| This Model is valid for Automotive grade 2 Temperature Range -40C<=Tc<=105C
| Valid for LPDDR4-4266 operation
| Part Number   VDD/VDDQ   Package   Architecture
| SCB11N4G160BF-04ZA2   1.1 +0.07/-0.04  BGA   4G bit x 16
[IBIS ver] 5.0
[File name]  usssn4g16ba2.ibs
[File Rev]  1.0
[Date]   October 8, 2023
[Source] Simulation of a silicon level SPICE model
[Notes]  IBIS Characteristics for I/O Buffer
  IBIS Model Revision History: Rev 1.0:
  2023-10-08 - IBIS model file initial creation
[Disclaimer]  The IBIS models are for modeling purpose only and are subject to change without any notice. UniIC is not
  responsible for any problems the models may cause.
[Copyright] Copyright 2023 UniIC Semiconductors Corp. All rights reserved
|   Component SCB11N4G160BF-04ZA2
[Component] SCB11N4G160BF-04ZA2
[Manufacturer] UniIC Semiconductors Corp.
[Package]
| variable   typ   min   max
R_pkg   0.750   0.698   0.832
L_pkg   1.500nH   1.330nH   1.720nH
C_pkg   0.630pF   0.579pF   0.668pF
[Pin]  signal_name   model_name   R_pin   L_pin   C_pin
A1   DNU   NC
A2   DNU   NC
A3   VSS   Gnd
A4   VDD2   Power
A5   ZQ0   NC
A8   NC   NC
A9   VDD2   Power
A10   VSS   Gnd
A11   DNU   NC
A12   DNU   NC
AA1   DNU   NC
AA2   NC   NC
AA3   VDDQ   Power
AA4   NC   NC
AA5   VDDQ   Power
AA8   VDDQ   Power
AA9   NC   NC
AA10   VDDQ   Power
AA11   NC   NC
AA12   DNU   NC
AB1   DNU   NC
AB2   DNU   NC
AB3   VSS   Gnd
AB4   VDD2   Power
AB5   VSS   Gnd
AB8   VSS   Gnd
AB9   VDD2   Power
AB10   VSS   Gnd
AB11   DNU   NC
AB12   DNU   NC
B1   DNU   NC
B2   DQ0_A   DQ   0.825   1.680nH   0.658pF
B3   VDDQ   Power
B4   DQ7_A   DQ   0.810   1.640nH   0.579pF
B5   VDDQ   Power
B8   VDDQ   Power
B9   DQ15_A   DQ   0.819   1.720nH   0.645pF
B10   VDDQ   Power
B11   DQ8_A   DQ   0.832   1.650nH   0.595pF
B12   DNU   NC
C1   VSS   Gnd
C2   DQ1_A   DQ   0.809   1.620nH   0.658pF
C3   DMI0_A   DQ   0.816   1.600nH   0.644pF
C4   DQ6_A   DQ   0.782   1.720nH   0.645pF
C5   VSS   Gnd
C8   VSS   Gnd
C9   DQ14_A   DQ   0.776   1.550nH   0.639pF
C10   DMI1_A   DQ   0.793   1.560nH   0.644pF
C11   DQ9_A   DQ   0.809   1.640nH   0.668pF
C12   VSS   Gnd
D1   VDDQ   Power
D2   VSS   Gnd
D3   DQS0_T_A   DQS   0.752   1.480nH   0.614pF
D4   VSS   Gnd
D5   VDDQ   Power
D8   VDDQ   Power
D9   VSS   Gnd
D10   DQS1_T_A   DQS   0.750   1.460nH   0.630pF
D11   VSS   Gnd
D12   VDDQ   Power
E1   VSS   Gnd
E2   DQ2_A   DQ   0.772   1.490nH   0.579pF
E3   DQS0_C_A   DQS   0.739   1.480nH   0.613pF
E4   DQ5_A   DQ   0.698   1.360nH   0.629pF
E5   VSS   Gnd
E8   VSS   Gnd
E9   DQ13_A   DQ   0.701   1.330nH   0.647pF
E10   DQS1_C_A   DQS   0.749   1.470nH   0.622pF
E11   DQ10_A   DQ   0.786   1.530nH   0.591pF
E12   VSS   Gnd
F1   VDD1   Power
F2   DQ3_A   DQ   0.748   1.480nH   0.582pF
F3   VDDQ   Power
F4   DQ4_A   DQ   0.740   1.430nH   0.640pF
F5   VDD2   Power
F8   VDD2   Power
F9   DQ12_A   DQ   0.751   1.420nH   0.664pF
F10   VDDQ   Power
F11   DQ11_A   DQ   0.765   1.520nH   0.562pF
F12   VDD1   Power
G1   VSS   Gnd
G2   ODTCA_A   RCV_RST_N
G3   VSS   Gnd
G4   VDD1   Power
G5   VSS   Gnd
G8   VSS   Gnd
G9   VDD1   Power
G10   VSS   Gnd
G11   NC   NC
G12   VSS   Gnd
H1   VDD2   Power
H2   CA0_A   CA   1.640   2.810nH   1.140pF
H3   NC   NC
H4   CS0_A   CA   1.170   2.210nH   0.905pF
H5   VDD2   Power
H8   VDD2   Power
H9   CA2_A   CA   1.550   2.690nH   1.150pF
H10   CA3_A   CA   1.570   2.740nH   1.120pF
H11   CA4_A   CA   1.600   2.780nH   1.160pF
H12   VDD2   Power
J1   VSS   Gnd
J2   CA1_A   CA   1.670   2.970nH   1.170pF
J3   VSS   Gnd
J4   CKE0_A   RCV_CKE   1.490   2.670nH   1.000pF
J5   NC   NC
J8   CKT_A   CLK   1.400   2.570nH   1.060pF
J9   CKC_A   CLK   1.420   2.610nH   1.070pF
J10   VSS   Gnd
J11   CA5_A   CA   1.710   2.940nH   1.200pF
J12   VSS   Gnd
K1   VDD2   Power
K2   VSS   Gnd
K3   VDD2   Power
K4   VSS   Gnd
K5   NC   NC
K8   NC   NC
K9   VSS   Gnd
K10   VDD2   Power
K11   VSS   Gnd
K12   VDD2   Power
N1   VDD2   Power
N2   VSS   Gnd
N3   VDD2   Power
N4   VSS   Gnd
N5   CS3_A   CA
N8   CKE3_A   RCV_CKE
N9   VSS   Gnd
N10   VDD2   Power
N11   VSS   Gnd
N12   VDD2   Power
P1   VSS   Gnd
P2   NC   NC
P3   VSS   Gnd
P4   NC   NC
P5   NC   NC
P8   NC   NC
P9   NC   NC
P10   VSS   Gnd
P11   NC   NC
P12   VSS   Gnd
R1   VDD2   Power
R2   NC   NC
R3   NC   NC
R4   NC   NC
R5   VDD2   Power
R8   VDD2   Power
R9   NC   NC
R10   NC   NC
R11   NC   NC
R12   VDD2   Power
T1   VSS   Gnd
T2   NC   NC
T3   VSS   Gnd
T4   VDD1   Power
T5   VSS   Gnd
T8   VSS   Gnd
T9   VDD1   Power
T10   VSS   Gnd
T11   RESET_N   RCV_RST_N
T12   VSS   Gnd
U1   VDD1   Power
U2   NC   NC
U3   VDDQ   Power
U4   NC   NC
U5   VDD2   Power
U8   VDD2   Power
U9   NC   NC
U10   VDDQ   Power
U11   NC   NC
U12   VDD1   Power
V1   VSS   Gnd
V2   NC   NC
V3   NC   NC
V4   NC   NC
V5   VSS   Gnd
V8   VSS   Gnd
V9   NC   NC
V10   NC   NC
V11   NC   NC
V12   VSS   Gnd
W1   VDDQ   Power
W2   VSS   Gnd
W3   NC   NC
W4   VSS   Gnd
W5   VDDQ   Power
W8   VDDQ   Power
W9   VSS   Gnd
W10   NC   NC
W11   VSS   Gnd
W12   VDDQ   Power
Y1   VSS   Gnd
Y2   NC   NC
Y3   NC   NC
Y4   NC   NC
Y5   VSS   Gnd
Y8   VSS   Gnd
Y9   NC   NC
Y10   NC   NC
Y11   NC   NC
Y12   VSS   Gnd
|IN   dq_in   dummy
|EN   dq_en   dummy
[Diff pin]  inv_pin  vdiff   tdelay_typ   tdelay_min   tdelay_max
D3   E3   0.160V   NA   NA   NA
D10   E10   0.160V   NA   NA   NA
J8   J9   0.160V   NA   NA   NA
[Model Selector] DQ
DQ_PU_PD_480_240_DRIVE_SOCODT240_VOH33  voh=vddq/3, 480 Ohm Pullup, 240 Ohm Pulldown,240ohm SOCODT
DQ_PU_PD_480_120_DRIVE_SOCODT240_VOH33  voh=vddq/3, 480 Ohm Pullup, 120 Ohm Pulldown,240ohm SOCODT
DQ_PU_PD_480_80_DRIVE_SOCODT240_VOH33  voh=vddq/3, 480 Ohm Pullup, 80 Ohm Pulldown,240ohm SOCODT
DQ_PU_PD_480_60_DRIVE_SOCODT240_VOH33  voh=vddq/3, 480 Ohm Pullup, 60 Ohm Pulldown,240ohm SOCODT
DQ_PU_PD_480_48_DRIVE_SOCODT240_VOH33  voh=vddq/3, 480 Ohm Pullup, 48 Ohm Pulldown,240ohm SOCODT
DQ_PU_PD_480_40_DRIVE_SOCODT240_VOH33  voh=vddq/3, 480 Ohm Pullup, 40 Ohm Pulldown,240ohm SOCODT
DQ_PU_PD_240_240_DRIVE_SOCODT120_VOH33  voh=vddq/3, 240 Ohm Pullup, 240 Ohm Pulldown,120ohm SOCODT
DQ_PU_PD_240_120_DRIVE_SOCODT120_VOH33  voh=vddq/3, 240 Ohm Pullup, 120 Ohm Pulldown,120ohm SOCODT
DQ_PU_PD_240_80_DRIVE_SOCODT120_VOH33  voh=vddq/3, 240 Ohm Pullup, 80 Ohm Pulldown,120ohm SOCODT
DQ_PU_PD_240_60_DRIVE_SOCODT120_VOH33  voh=vddq/3, 240 Ohm Pullup, 60 Ohm Pulldown,120ohm SOCODT
DQ_PU_PD_240_48_DRIVE_SOCODT120_VOH33  voh=vddq/3, 240 Ohm Pullup, 48 Ohm Pulldown,120ohm SOCODT
DQ_PU_PD_240_40_DRIVE_SOCODT120_VOH33  voh=vddq/3, 240 Ohm Pullup, 40 Ohm Pulldown,120ohm SOCODT
DQ_PU_PD_160_240_DRIVE_SOCODT80_VOH33  voh=vddq/3, 160 Ohm Pullup, 240 Ohm Pulldown,80ohm SOCODT
DQ_PU_PD_160_120_DRIVE_SOCODT80_VOH33  voh=vddq/3, 160 Ohm Pullup, 120 Ohm Pulldown,80ohm SOCODT
DQ_PU_PD_160_80_DRIVE_SOCODT80_VOH33  voh=vddq/3, 160 Ohm Pullup, 80 Ohm Pulldown,80ohm SOCODT
DQ_PU_PD_160_60_DRIVE_SOCODT80_VOH33  voh=vddq/3, 160 Ohm Pullup, 60 Ohm Pulldown,80ohm SOCODT
DQ_PU_PD_160_48_DRIVE_SOCODT80_VOH33  voh=vddq/3, 160 Ohm Pullup, 48 Ohm Pulldown,80ohm SOCODT
DQ_PU_PD_160_40_DRIVE_SOCODT80_VOH33  voh=vddq/3, 160 Ohm Pullup, 40 Ohm Pulldown,80ohm SOCODT
DQ_PU_PD_120_240_DRIVE_SOCODT60_VOH33  voh=vddq/3, 120 Ohm Pullup, 240 Ohm Pulldown,60ohm SOCODT
DQ_PU_PD_120_120_DRIVE_SOCODT60_VOH33  voh=vddq/3, 120 Ohm Pullup, 120 Ohm Pulldown,60ohm SOCODT
DQ_PU_PD_120_80_DRIVE_SOCODT60_VOH33  voh=vddq/3, 120 Ohm Pullup, 80 Ohm Pulldown,60ohm SOCODT
DQ_PU_PD_120_60_DRIVE_SOCODT60_VOH33  voh=vddq/3, 120 Ohm Pullup, 60 Ohm Pulldown,60ohm SOCODT
DQ_PU_PD_120_48_DRIVE_SOCODT60_VOH33  voh=vddq/3, 120 Ohm Pullup, 48 Ohm Pulldown,60ohm SOCODT
DQ_PU_PD_120_40_DRIVE_SOCODT60_VOH33  voh=vddq/3, 120 Ohm Pullup, 40 Ohm Pulldown,60ohm SOCODT
DQ_PU_PD_96_240_DRIVE_SOCODT48_VOH33  voh=vddq/3, 96 Ohm Pullup, 240 Ohm Pulldown,48ohm SOCODT
DQ_PU_PD_96_120_DRIVE_SOCODT48_VOH33  voh=vddq/3, 96 Ohm Pullup, 120 Ohm Pulldown,48ohm SOCODT
DQ_PU_PD_96_80_DRIVE_SOCODT48_VOH33  voh=vddq/3, 96 Ohm Pullup, 80 Ohm Pulldown,48ohm SOCODT
DQ_PU_PD_96_60_DRIVE_SOCODT48_VOH33  voh=vddq/3, 96 Ohm Pullup, 60 Ohm Pulldown,48ohm SOCODT
DQ_PU_PD_96_48_DRIVE_SOCODT48_VOH33  voh=vddq/3, 96 Ohm Pullup, 48 Ohm Pulldown,48ohm SOCODT
DQ_PU_PD_96_40_DRIVE_SOCODT48_VOH33  voh=vddq/3, 96 Ohm Pullup, 40 Ohm Pulldown,48ohm SOCODT
DQ_PU_PD_80_240_DRIVE_SOCODT40_VOH33  voh=vddq/3, 80 Ohm Pullup, 240 Ohm Pulldown,SOCODT disable OR 40ohm SOCODT
DQ_PU_PD_80_120_DRIVE_SOCODT40_VOH33  voh=vddq/3, 80 Ohm Pullup, 120 Ohm Pulldown,SOCODT disable OR 40ohm SOCODT
DQ_PU_PD_80_80_DRIVE_SOCODT40_VOH33  voh=vddq/3, 80 Ohm Pullup, 80 Ohm Pulldown,SOCODT disable OR 40ohm SOCODT
DQ_PU_PD_80_60_DRIVE_SOCODT40_VOH33  voh=vddq/3, 80 Ohm Pullup, 60 Ohm Pulldown,SOCODT disable OR 40ohm SOCODT
DQ_PU_PD_80_48_DRIVE_SOCODT40_VOH33  voh=vddq/3, 80 Ohm Pullup, 48 Ohm Pulldown,SOCODT disable OR 40ohm SOCODT
DQ_PU_PD_80_40_DRIVE_SOCODT40_VOH33  voh=vddq/3, 80 Ohm Pullup, 40 Ohm Pulldown,SOCODT disable OR 40ohm SOCODT
DQ_PU_PD_120_240_DRIVE_SOCODT80_VOH40  voh=vddq/2.5, 120 Ohm Pullup, 240 Ohm Pulldown,SOCODT disable OR 80ohm SOCODT
DQ_PU_PD_120_120_DRIVE_SOCODT80_VOH40  voh=vddq/2.5, 120 Ohm Pullup, 120 Ohm Pulldown,SOCODT disable OR 80ohm SOCODT
DQ_PU_PD_120_80_DRIVE_SOCODT80_VOH40  voh=vddq/2.5, 120 Ohm Pullup, 80 Ohm Pulldown,SOCODT disable OR 80ohm SOCODT
DQ_PU_PD_120_60_DRIVE_SOCODT80_VOH40  voh=vddq/2.5, 120 Ohm Pullup, 60 Ohm Pulldown,SOCODT disable OR 80ohm SOCODT
DQ_PU_PD_120_48_DRIVE_SOCODT80_VOH40  voh=vddq/2.5, 120 Ohm Pullup, 48 Ohm Pulldown,SOCODT disable OR 80ohm SOCODT
DQ_PU_PD_120_40_DRIVE_SOCODT80_VOH40  voh=vddq/2.5, 120 Ohm Pullup, 40 Ohm Pulldown,SOCODT disable OR 80ohm SOCODT
DQ_PU_PD_180_240_DRIVE_SOCODT120_VOH40  voh=vddq/2.5, 180 Ohm Pullup, 240 Ohm Pulldown,120ohm SOCODT
DQ_PU_PD_180_120_DRIVE_SOCODT120_VOH40  voh=vddq/2.5, 180 Ohm Pullup, 120 Ohm Pulldown,120ohm SOCODT
DQ_PU_PD_180_80_DRIVE_SOCODT120_VOH40  voh=vddq/2.5, 180 Ohm Pullup, 80 Ohm Pulldown,120ohm SOCODT
DQ_PU_PD_180_60_DRIVE_SOCODT120_VOH40  voh=vddq/2.5, 180 Ohm Pullup, 60 Ohm Pulldown,120ohm SOCODT
DQ_PU_PD_180_48_DRIVE_SOCODT120_VOH40  voh=vddq/2.5, 180 Ohm Pullup, 48 Ohm Pulldown,120ohm SOCODT
DQ_PU_PD_180_40_DRIVE_SOCODT120_VOH40  voh=vddq/2.5, 180 Ohm Pullup, 40 Ohm Pulldown,120ohm SOCODT
DQ_PU_PD_360_240_DRIVE_SOCODT240_VOH40  voh=vddq/2.5, 360 Ohm Pullup, 240 Ohm Pulldown,240ohm SOCODT
DQ_PU_PD_360_120_DRIVE_SOCODT240_VOH40  voh=vddq/2.5, 360 Ohm Pullup, 120 Ohm Pulldown,240ohm SOCODT
DQ_PU_PD_360_80_DRIVE_SOCODT240_VOH40  voh=vddq/2.5, 360 Ohm Pullup, 80 Ohm Pulldown,240ohm SOCODT
DQ_PU_PD_360_60_DRIVE_SOCODT240_VOH40  voh=vddq/2.5, 360 Ohm Pullup, 60 Ohm Pulldown,240ohm SOCODT
DQ_PU_PD_360_48_DRIVE_SOCODT240_VOH40  voh=vddq/2.5, 360 Ohm Pullup, 48 Ohm Pulldown,240ohm SOCODT
DQ_PU_PD_360_40_DRIVE_SOCODT240_VOH40  voh=vddq/2.5, 360 Ohm Pullup, 40 Ohm Pulldown,240ohm SOCODT
DQ_ODTOFF  DQ Type input, ODT off for DQ_RCV
DQ_ODT40_VOH33  voh=vddq/3, DQ Type input, ODT 40 for DQ_RCV
DQ_ODT48_VOH33  voh=vddq/3, DQ Type input, ODT 48 for DQ_RCV
DQ_ODT60_VOH33  voh=vddq/3, DQ Type input, ODT 60 for DQ_RCV
DQ_ODT80_VOH33  voh=vddq/3, DQ Type input, ODT 80 for DQ_RCV
DQ_ODT120_VOH33  voh=vddq/3, DQ Type input, ODT 120 for DQ_RCV
DQ_ODT240_VOH33  voh=vddq/3, DQ Type input, ODT 240 for DQ_RCV
DQ_ODT40_VOH40  voh=vddq/2.5, DQ Type input, ODT 40 for DQ_RCV
DQ_ODT48_VOH40  voh=vddq/2.5, DQ Type input, ODT 48 for DQ_RCV
DQ_ODT60_VOH40  voh=vddq/2.5, DQ Type input, ODT 60 for DQ_RCV
DQ_ODT80_VOH40  voh=vddq/2.5, DQ Type input, ODT 80 for DQ_RCV
DQ_ODT120_VOH40  voh=vddq/2.5, DQ Type input, ODT 120 for DQ_RCV
DQ_ODT240_VOH40  voh=vddq/2.5, DQ Type input, ODT 240 for DQ_RCV
[Model Selector] DQS
DQS_PU_PD_480_240_DRIVE_SOCODT240_VOH33  voh=vddq/3, 480 Ohm Pullup, 240 Ohm Pulldown,240ohm SOCODT
DQS_PU_PD_480_120_DRIVE_SOCODT240_VOH33  voh=vddq/3, 480 Ohm Pullup, 120 Ohm Pulldown,240ohm SOCODT
DQS_PU_PD_480_80_DRIVE_SOCODT240_VOH33  voh=vddq/3, 480 Ohm Pullup, 80 Ohm Pulldown,240ohm SOCODT
DQS_PU_PD_480_60_DRIVE_SOCODT240_VOH33  voh=vddq/3, 480 Ohm Pullup, 60 Ohm Pulldown,240ohm SOCODT
DQS_PU_PD_480_48_DRIVE_SOCODT240_VOH33  voh=vddq/3, 480 Ohm Pullup, 48 Ohm Pulldown,240ohm SOCODT
DQS_PU_PD_480_40_DRIVE_SOCODT240_VOH33  voh=vddq/3, 480 Ohm Pullup, 40 Ohm Pulldown,240ohm SOCODT
DQS_PU_PD_240_240_DRIVE_SOCODT120_VOH33  voh=vddq/3, 240 Ohm Pullup, 240 Ohm Pulldown,120ohm SOCODT
DQS_PU_PD_240_120_DRIVE_SOCODT120_VOH33  voh=vddq/3, 240 Ohm Pullup, 120 Ohm Pulldown,120ohm SOCODT
DQS_PU_PD_240_80_DRIVE_SOCODT120_VOH33  voh=vddq/3, 240 Ohm Pullup, 80 Ohm Pulldown,120ohm SOCODT
DQS_PU_PD_240_60_DRIVE_SOCODT120_VOH33  voh=vddq/3, 240 Ohm Pullup, 60 Ohm Pulldown,120ohm SOCODT
DQS_PU_PD_240_48_DRIVE_SOCODT120_VOH33  voh=vddq/3, 240 Ohm Pullup, 48 Ohm Pulldown,120ohm SOCODT
DQS_PU_PD_240_40_DRIVE_SOCODT120_VOH33  voh=vddq/3, 240 Ohm Pullup, 40 Ohm Pulldown,120ohm SOCODT
DQS_PU_PD_160_240_DRIVE_SOCODT80_VOH33  voh=vddq/3, 160 Ohm Pullup, 240 Ohm Pulldown,80ohm SOCODT
DQS_PU_PD_160_120_DRIVE_SOCODT80_VOH33  voh=vddq/3, 160 Ohm Pullup, 120 Ohm Pulldown,80ohm SOCODT
DQS_PU_PD_160_80_DRIVE_SOCODT80_VOH33  voh=vddq/3, 160 Ohm Pullup, 80 Ohm Pulldown,80ohm SOCODT
DQS_PU_PD_160_60_DRIVE_SOCODT80_VOH33  voh=vddq/3, 160 Ohm Pullup, 60 Ohm Pulldown,80ohm SOCODT
DQS_PU_PD_160_48_DRIVE_SOCODT80_VOH33  voh=vddq/3, 160 Ohm Pullup, 48 Ohm Pulldown,80ohm SOCODT
DQS_PU_PD_160_40_DRIVE_SOCODT80_VOH33  voh=vddq/3, 160 Ohm Pullup, 40 Ohm Pulldown,80ohm SOCODT
DQS_PU_PD_120_240_DRIVE_SOCODT60_VOH33  voh=vddq/3, 120 Ohm Pullup, 240 Ohm Pulldown,60ohm SOCODT
DQS_PU_PD_120_120_DRIVE_SOCODT60_VOH33  voh=vddq/3, 120 Ohm Pullup, 120 Ohm Pulldown,60ohm SOCODT
DQS_PU_PD_120_80_DRIVE_SOCODT60_VOH33  voh=vddq/3, 120 Ohm Pullup, 80 Ohm Pulldown,60ohm SOCODT
DQS_PU_PD_120_60_DRIVE_SOCODT60_VOH33  voh=vddq/3, 120 Ohm Pullup, 60 Ohm Pulldown,60ohm SOCODT
DQS_PU_PD_120_48_DRIVE_SOCODT60_VOH33  voh=vddq/3, 120 Ohm Pullup, 48 Ohm Pulldown,60ohm SOCODT
DQS_PU_PD_120_40_DRIVE_SOCODT60_VOH33  voh=vddq/3, 120 Ohm Pullup, 40 Ohm Pulldown,60ohm SOCODT
DQS_PU_PD_96_240_DRIVE_SOCODT48_VOH33  voh=vddq/3, 96 Ohm Pullup, 240 Ohm Pulldown,48ohm SOCODT
DQS_PU_PD_96_120_DRIVE_SOCODT48_VOH33  voh=vddq/3, 96 Ohm Pullup, 120 Ohm Pulldown,48ohm SOCODT
DQS_PU_PD_96_80_DRIVE_SOCODT48_VOH33  voh=vddq/3, 96 Ohm Pullup, 80 Ohm Pulldown,48ohm SOCODT
DQS_PU_PD_96_60_DRIVE_SOCODT48_VOH33  voh=vddq/3, 96 Ohm Pullup, 60 Ohm Pulldown,48ohm SOCODT
DQS_PU_PD_96_48_DRIVE_SOCODT48_VOH33  voh=vddq/3, 96 Ohm Pullup, 48 Ohm Pulldown,48ohm SOCODT
DQS_PU_PD_96_40_DRIVE_SOCODT48_VOH33  voh=vddq/3, 96 Ohm Pullup, 40 Ohm Pulldown,48ohm SOCODT
DQS_PU_PD_80_240_DRIVE_SOCODT40_VOH33  voh=vddq/3, 80 Ohm Pullup, 240 Ohm Pulldown,SOCODT disable OR 40ohm SOCODT
DQS_PU_PD_80_120_DRIVE_SOCODT40_VOH33  voh=vddq/3, 80 Ohm Pullup, 120 Ohm Pulldown,SOCODT disable OR 40ohm SOCODT
DQS_PU_PD_80_80_DRIVE_SOCODT40_VOH33  voh=vddq/3, 80 Ohm Pullup, 80 Ohm Pulldown,SOCODT disable OR 40ohm SOCODT
DQS_PU_PD_80_60_DRIVE_SOCODT40_VOH33  voh=vddq/3, 80 Ohm Pullup, 60 Ohm Pulldown,SOCODT disable OR 40ohm SOCODT
DQS_PU_PD_80_48_DRIVE_SOCODT40_VOH33  voh=vddq/3, 80 Ohm Pullup, 48 Ohm Pulldown,SOCODT disable OR 40ohm SOCODT
DQS_PU_PD_80_40_DRIVE_SOCODT40_VOH33  voh=vddq/3, 80 Ohm Pullup, 40 Ohm Pulldown,SOCODT disable OR 40ohm SOCODT
DQS_PU_PD_120_240_DRIVE_SOCODT80_VOH40  voh=vddq/2.5, 120 Ohm Pullup, 240 Ohm Pulldown,SOCODT disable OR 80ohm SOCODT
DQS_PU_PD_120_120_DRIVE_SOCODT80_VOH40  voh=vddq/2.5, 120 Ohm Pullup, 120 Ohm Pulldown,SOCODT disable OR 80ohm SOCODT
DQS_PU_PD_120_80_DRIVE_SOCODT80_VOH40  voh=vddq/2.5, 120 Ohm Pullup, 80 Ohm Pulldown,SOCODT disable OR 80ohm SOCODT
DQS_PU_PD_120_60_DRIVE_SOCODT80_VOH40  voh=vddq/2.5, 120 Ohm Pullup, 60 Ohm Pulldown,SOCODT disable OR 80ohm SOCODT
DQS_PU_PD_120_48_DRIVE_SOCODT80_VOH40  voh=vddq/2.5, 120 Ohm Pullup, 48 Ohm Pulldown,SOCODT disable OR 80ohm SOCODT
DQS_PU_PD_120_40_DRIVE_SOCODT80_VOH40  voh=vddq/2.5, 120 Ohm Pullup, 40 Ohm Pulldown,SOCODT disable OR 80ohm SOCODT
DQS_PU_PD_180_240_DRIVE_SOCODT120_VOH40  voh=vddq/2.5, 180 Ohm Pullup, 240 Ohm Pulldown,120ohm SOCODT
DQS_PU_PD_180_120_DRIVE_SOCODT120_VOH40  voh=vddq/2.5, 180 Ohm Pullup, 120 Ohm Pulldown,120ohm SOCODT
DQS_PU_PD_180_80_DRIVE_SOCODT120_VOH40  voh=vddq/2.5, 180 Ohm Pullup, 80 Ohm Pulldown,120ohm SOCODT
DQS_PU_PD_180_60_DRIVE_SOCODT120_VOH40  voh=vddq/2.5, 180 Ohm Pullup, 60 Ohm Pulldown,120ohm SOCODT
DQS_PU_PD_180_48_DRIVE_SOCODT120_VOH40  voh=vddq/2.5, 180 Ohm Pullup, 48 Ohm Pulldown,120ohm SOCODT
DQS_PU_PD_180_40_DRIVE_SOCODT120_VOH40  voh=vddq/2.5, 180 Ohm Pullup, 40 Ohm Pulldown,120ohm SOCODT
DQS_PU_PD_360_240_DRIVE_SOCODT240_VOH40  voh=vddq/2.5, 360 Ohm Pullup, 240 Ohm Pulldown,240ohm SOCODT
DQS_PU_PD_360_120_DRIVE_SOCODT240_VOH40  voh=vddq/2.5, 360 Ohm Pullup, 120 Ohm Pulldown,240ohm SOCODT
DQS_PU_PD_360_80_DRIVE_SOCODT240_VOH40  voh=vddq/2.5, 360 Ohm Pullup, 80 Ohm Pulldown,240ohm SOCODT
DQS_PU_PD_360_60_DRIVE_SOCODT240_VOH40  voh=vddq/2.5, 360 Ohm Pullup, 60 Ohm Pulldown,240ohm SOCODT
DQS_PU_PD_360_48_DRIVE_SOCODT240_VOH40  voh=vddq/2.5, 360 Ohm Pullup, 48 Ohm Pulldown,240ohm SOCODT
DQS_PU_PD_360_40_DRIVE_SOCODT240_VOH40  voh=vddq/2.5, 360 Ohm Pullup, 40 Ohm Pulldown,240ohm SOCODT
DQS_ODTOFF  DQS Type input, ODT off for DQS_RCV
DQS_ODT40_VOH33  voh=vddq/3, DQS Type input, ODT 40 for DQS_RCV
DQS_ODT48_VOH33  voh=vddq/3, DQS Type input, ODT 48 for DQS_RCV
DQS_ODT60_VOH33  voh=vddq/3, DQS Type input, ODT 60 for DQS_RCV
DQS_ODT80_VOH33  voh=vddq/3, DQS Type input, ODT 80 for DQS_RCV
DQS_ODT120_VOH33  voh=vddq/3, DQS Type input, ODT 120 for DQS_RCV
DQS_ODT240_VOH33  voh=vddq/3, DQS Type input, ODT 240 for DQS_RCV
DQS_ODT40_VOH40  voh=vddq/2.5, DQS Type input, ODT 40 for DQS_RCV
DQS_ODT48_VOH40  voh=vddq/2.5, DQS Type input, ODT 48 for DQS_RCV
DQS_ODT60_VOH40  voh=vddq/2.5, DQS Type input, ODT 60 for DQS_RCV
DQS_ODT80_VOH40  voh=vddq/2.5, DQS Type input, ODT 80 for DQS_RCV
DQS_ODT120_VOH40  voh=vddq/2.5, DQS Type input, ODT 120 for DQS_RCV
DQS_ODT240_VOH40  voh=vddq/2.5, DQS Type input, ODT 240 for DQS_RCV
[Model Selector] CA
CA_ODTOFF  CA/CS_N Type input, ODT off for CA_RCV
CA_ODT40_VOH33  voh=vddq/3, CA/CS_N Type input, 40 ohm ODT for CA_RCV
CA_ODT48_VOH33  voh=vddq/3, CA/CS_N Type input, 48 ohm ODT for CA_RCV
CA_ODT60_VOH33  voh=vddq/3, CA/CS_N Type input, 60 ohm ODT for CA_RCV
CA_ODT80_VOH33  voh=vddq/3, CA/CS_N Type input, 80 ohm ODT for CA_RCV
CA_ODT120_VOH33  voh=vddq/3, CA/CS_N Type input, 120 ohm ODT for CA_RCV
CA_ODT240_VOH33  voh=vddq/3, CA/CS_N Type input, 240 ohm ODT for CA_RCV
CA_ODT40_VOH40  voh=vddq/2.5, CA/CS_N Type input, 40 ohm ODT for CA_RCV
CA_ODT48_VOH40  voh=vddq/2.5, CA/CS_N Type input, 48 ohm ODT for CA_RCV
CA_ODT60_VOH40  voh=vddq/2.5, CA/CS_N Type input, 60 ohm ODT for CA_RCV
CA_ODT80_VOH40  voh=vddq/2.5, CA/CS_N Type input, 80 ohm ODT for CA_RCV
CA_ODT120_VOH40  voh=vddq/2.5, CA/CS_N Type input, 120 ohm ODT for CA_RCV
CA_ODT240_VOH40  voh=vddq/2.5, CA/CS_N Type input, 240 ohm ODT for CA_RCV
[Model Selector] CLK
CLK_ODTOFF  CLK Type input, ODT off for CLK_RCV
CLK_ODT40_VOH33  voh=vddq/3, CLK Type input, 40 ohm ODT for CLK_RCV
CLK_ODT48_VOH33  voh=vddq/3, CLK Type input, 48 ohm ODT for CLK_RCV
CLK_ODT60_VOH33  voh=vddq/3, CLK Type input, 60 ohm ODT for CLK_RCV
CLK_ODT80_VOH33  voh=vddq/3, CLK Type input, 80 ohm ODT for CLK_RCV
CLK_ODT120_VOH33  voh=vddq/3, CLK Type input, 120 ohm ODT for CLK_RCV
CLK_ODT240_VOH33  voh=vddq/3, CLK Type input, 240 ohm ODT for CLK_RCV
CLK_ODT40_VOH40  voh=vddq/2.5, CLK Type input, 40 ohm ODT for CLK_RCV
CLK_ODT48_VOH40  voh=vddq/2.5, CLK Type input, 48 ohm ODT for CLK_RCV
CLK_ODT60_VOH40  voh=vddq/2.5, CLK Type input, 60 ohm ODT for CLK_RCV
CLK_ODT80_VOH40  voh=vddq/2.5, CLK Type input, 80 ohm ODT for CLK_RCV
CLK_ODT120_VOH40  voh=vddq/2.5, CLK Type input, 120 ohm ODT for CLK_RCV
CLK_ODT240_VOH40  voh=vddq/2.5, CLK Type input, 240 ohm ODT for CLK_RCV
| Models and submodels in the file (186): DQ_PU_PD_480_240_DRIVE_SOCODT240_VOH33 (I/O), DQ_PU_PD_480_120_DRIVE_SOCODT240_VOH33 (I/O), DQ_PU_PD_480_80_DRIVE_SOCODT240_VOH33 (I/O), DQ_PU_PD_480_60_DRIVE_SOCODT240_VOH33 (I/O), DQ_PU_PD_480_48_DRIVE_SOCODT240_VOH33 (I/O), DQ_PU_PD_480_40_DRIVE_SOCODT240_VOH33 (I/O), DQ_PU_PD_240_240_DRIVE_SOCODT120_VOH33 (I/O), DQ_PU_PD_240_120_DRIVE_SOCODT120_VOH33 (I/O), DQ_PU_PD_240_80_DRIVE_SOCODT120_VOH33 (I/O), DQ_PU_PD_240_60_DRIVE_SOCODT120_VOH33 (I/O), DQ_PU_PD_240_48_DRIVE_SOCODT120_VOH33 (I/O), DQ_PU_PD_240_40_DRIVE_SOCODT120_VOH33 (I/O), DQ_PU_PD_160_240_DRIVE_SOCODT80_VOH33 (I/O), DQ_PU_PD_160_120_DRIVE_SOCODT80_VOH33 (I/O), DQ_PU_PD_160_80_DRIVE_SOCODT80_VOH33 (I/O), DQ_PU_PD_160_60_DRIVE_SOCODT80_VOH33 (I/O), DQ_PU_PD_160_48_DRIVE_SOCODT80_VOH33 (I/O), DQ_PU_PD_160_40_DRIVE_SOCODT80_VOH33 (I/O), DQ_PU_PD_120_240_DRIVE_SOCODT60_VOH33 (I/O), DQ_PU_PD_120_120_DRIVE_SOCODT60_VOH33 (I/O), DQ_PU_PD_120_80_DRIVE_SOCODT60_VOH33 (I/O), DQ_PU_PD_120_60_DRIVE_SOCODT60_VOH33 (I/O), DQ_PU_PD_120_48_DRIVE_SOCODT60_VOH33 (I/O), DQ_PU_PD_120_40_DRIVE_SOCODT60_VOH33 (I/O), DQ_PU_PD_96_240_DRIVE_SOCODT48_VOH33 (I/O), DQ_PU_PD_96_120_DRIVE_SOCODT48_VOH33 (I/O), DQ_PU_PD_96_80_DRIVE_SOCODT48_VOH33 (I/O), DQ_PU_PD_96_60_DRIVE_SOCODT48_VOH33 (I/O), DQ_PU_PD_96_48_DRIVE_SOCODT48_VOH33 (I/O), DQ_PU_PD_96_40_DRIVE_SOCODT48_VOH33 (I/O), DQ_PU_PD_80_240_DRIVE_SOCODT40_VOH33 (I/O), DQ_PU_PD_80_120_DRIVE_SOCODT40_VOH33 (I/O), DQ_PU_PD_80_80_DRIVE_SOCODT40_VOH33 (I/O), DQ_PU_PD_80_60_DRIVE_SOCODT40_VOH33 (I/O), DQ_PU_PD_80_48_DRIVE_SOCODT40_VOH33 (I/O), DQ_PU_PD_80_40_DRIVE_SOCODT40_VOH33 (I/O), DQ_PU_PD_360_240_DRIVE_SOCODT240_VOH40 (I/O), DQ_PU_PD_360_120_DRIVE_SOCODT240_VOH40 (I/O), DQ_PU_PD_360_80_DRIVE_SOCODT240_VOH40 (I/O), DQ_PU_PD_360_60_DRIVE_SOCODT240_VOH40 (I/O), DQ_PU_PD_360_48_DRIVE_SOCODT240_VOH40 (I/O), DQ_PU_PD_360_40_DRIVE_SOCODT240_VOH40 (I/O), DQ_PU_PD_180_240_DRIVE_SOCODT120_VOH40 (I/O), DQ_PU_PD_180_120_DRIVE_SOCODT120_VOH40 (I/O), DQ_PU_PD_180_80_DRIVE_SOCODT120_VOH40 (I/O), DQ_PU_PD_180_60_DRIVE_SOCODT120_VOH40 (I/O), DQ_PU_PD_180_48_DRIVE_SOCODT120_VOH40 (I/O), DQ_PU_PD_180_40_DRIVE_SOCODT120_VOH40 (I/O), DQ_PU_PD_120_240_DRIVE_SOCODT80_VOH40 (I/O), DQ_PU_PD_120_120_DRIVE_SOCODT80_VOH40 (I/O), DQ_PU_PD_120_80_DRIVE_SOCODT80_VOH40 (I/O), DQ_PU_PD_120_60_DRIVE_SOCODT80_VOH40 (I/O), DQ_PU_PD_120_48_DRIVE_SOCODT80_VOH40 (I/O), DQ_PU_PD_120_40_DRIVE_SOCODT80_VOH40 (I/O), DQS_PU_PD_480_240_DRIVE_SOCODT240_VOH33 (I/O), DQS_PU_PD_480_120_DRIVE_SOCODT240_VOH33 (I/O), DQS_PU_PD_480_80_DRIVE_SOCODT240_VOH33 (I/O), DQS_PU_PD_480_60_DRIVE_SOCODT240_VOH33 (I/O), DQS_PU_PD_480_48_DRIVE_SOCODT240_VOH33 (I/O), DQS_PU_PD_480_40_DRIVE_SOCODT240_VOH33 (I/O), DQS_PU_PD_240_240_DRIVE_SOCODT120_VOH33 (I/O), DQS_PU_PD_240_120_DRIVE_SOCODT120_VOH33 (I/O), DQS_PU_PD_240_80_DRIVE_SOCODT120_VOH33 (I/O), DQS_PU_PD_240_60_DRIVE_SOCODT120_VOH33 (I/O), DQS_PU_PD_240_48_DRIVE_SOCODT120_VOH33 (I/O), DQS_PU_PD_240_40_DRIVE_SOCODT120_VOH33 (I/O), DQS_PU_PD_160_240_DRIVE_SOCODT80_VOH33 (I/O), DQS_PU_PD_160_120_DRIVE_SOCODT80_VOH33 (I/O), DQS_PU_PD_160_80_DRIVE_SOCODT80_VOH33 (I/O), DQS_PU_PD_160_60_DRIVE_SOCODT80_VOH33 (I/O), DQS_PU_PD_160_48_DRIVE_SOCODT80_VOH33 (I/O), DQS_PU_PD_160_40_DRIVE_SOCODT80_VOH33 (I/O), DQS_PU_PD_120_240_DRIVE_SOCODT60_VOH33 (I/O), DQS_PU_PD_120_120_DRIVE_SOCODT60_VOH33 (I/O), DQS_PU_PD_120_80_DRIVE_SOCODT60_VOH33 (I/O), DQS_PU_PD_120_60_DRIVE_SOCODT60_VOH33 (I/O), DQS_PU_PD_120_48_DRIVE_SOCODT60_VOH33 (I/O), DQS_PU_PD_120_40_DRIVE_SOCODT60_VOH33 (I/O), DQS_PU_PD_96_240_DRIVE_SOCODT48_VOH33 (I/O), DQS_PU_PD_96_120_DRIVE_SOCODT48_VOH33 (I/O)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
